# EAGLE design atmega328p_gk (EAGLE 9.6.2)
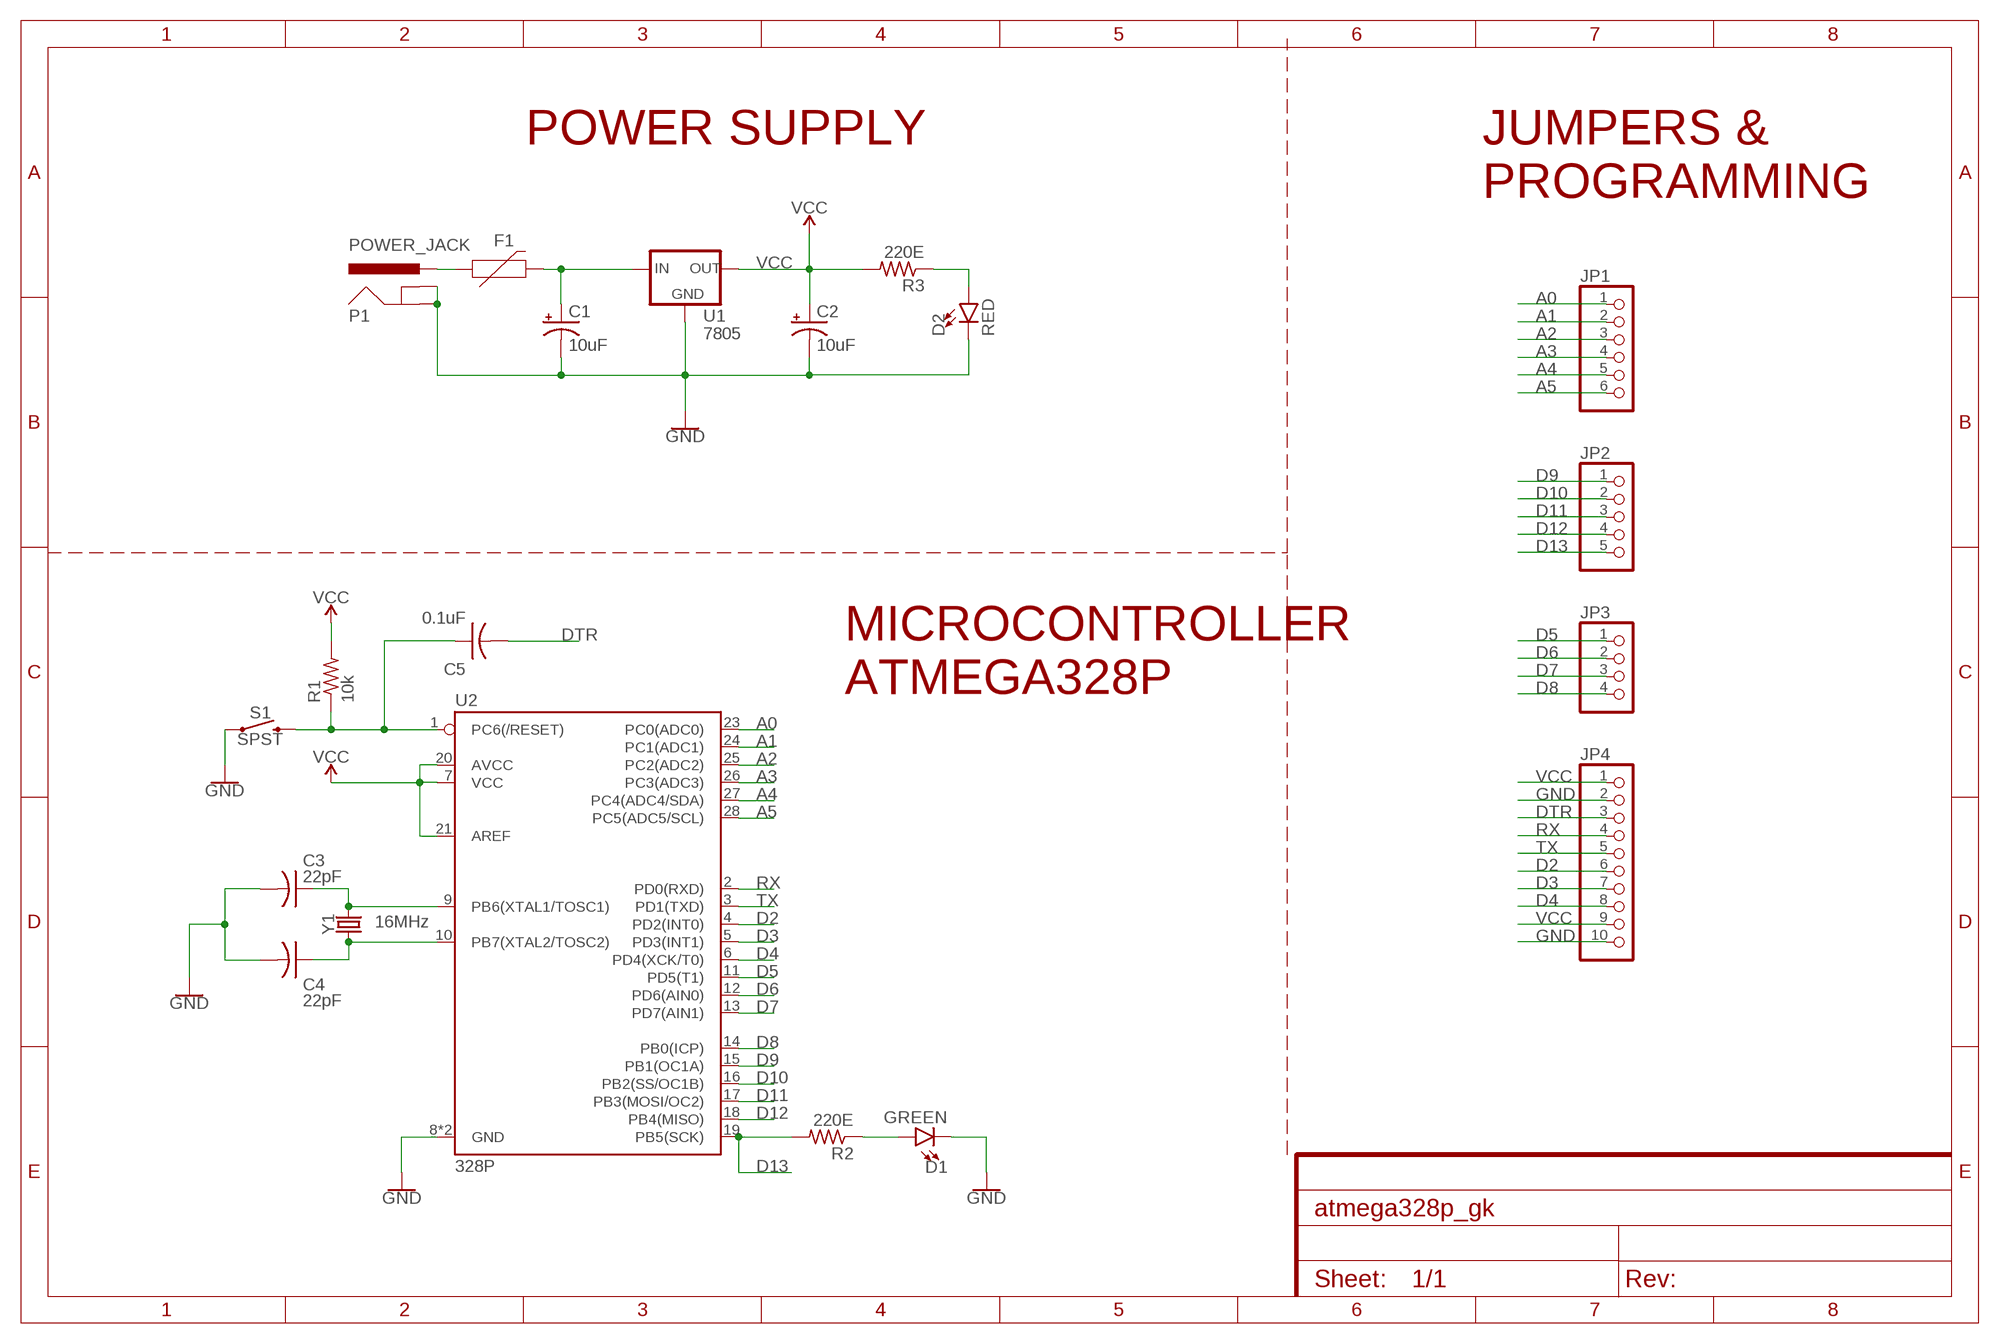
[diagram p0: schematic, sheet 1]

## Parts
C1  10uF  CPOL-USE2,5-6E  [E2,5-6E]
C2  10uF  CPOL-USE2,5-6E  [E2,5-6E]
C3  22pF  C-US025-024X044  [C025-024X044]
C4  22pF  C-US025-024X044  [C025-024X044]
C5  0.1uF  C-US025-024X044  [C025-024X044]
D1  GREEN  LED-GREEN0603  [LED-0603]
D2  RED  LED-RED0603  [LED-0603]
F1  PPTC_16V_2.5A  [1812]
JP1  PINHD-1X6  [1X06]
JP2  PINHD-1X5  [1X05]
JP3  PINHD-1X4  [1X04]
JP4  PINHD-1X10  [1X10]
P1  POWER_JACK  POWER_JACKPTH_LOCK  [POWER_JACK_PTH_LOCK]
R1  10k  R-US_0204/7  [0204/7]
R2  220E  R-US_0204/7  [0204/7]
R3  220E  R-US_0204/7  [0204/7]
S1  SPST  MOMENTARY-SWITCH-SPST-PTH-6.0MM  [TACTILE_SWITCH_PTH_6.0MM]
U1  7805  78XXS  [78XXS]
U2  328P  ATMEGA328P_PDIP  [DIP28]
Y1  16MHz  CRYSTAL-16MHZPTH-HC49US  [HC49US]

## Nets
A0: JP1.1 U2.23(PC0(ADC0))
A1: JP1.2 U2.24(PC1(ADC1))
A2: JP1.3 U2.25(PC2(ADC2))
A3: JP1.4 U2.26(PC3(ADC3))
A4: JP1.5 U2.27(PC4(ADC4/SDA))
A5: JP1.6 U2.28(PC5(ADC5/SCL))
D2: JP4.6 U2.4(PD2(INT0))
D3: JP4.7 U2.5(PD3(INT1))
D4: JP4.8 U2.6(PD4(XCK/T0))
D5: JP3.1 U2.11(PD5(T1))
D6: JP3.2 U2.12(PD6(AIN0))
D7: JP3.3 U2.13(PD7(AIN1))
D8: JP3.4 U2.14(PB0(ICP))
D9: JP2.1 U2.15(PB1(OC1A))
D10: JP2.2 U2.16(PB2(SS/OC1B))
D11: JP2.3 U2.17(PB3(MOSI/OC2))
D12: JP2.4 U2.18(PB4(MISO))
D13: JP2.5 R2.2 U2.19(PB5(SCK))
DTR: C5.2 JP4.3
GND: C1.- C2.- C3.2 C4.2 D1.C D2.C JP4.2 JP4.10 P1.GND P1.GNDBREAK S1.1 U1.GND U2.8(GND) U2.22(GND)
N$1: C1.+ F1.2 U1.IN
N$2: C3.1 U2.9(PB6(XTAL1/TOSC1)) Y1.2
N$3: C4.1 U2.10(PB7(XTAL2/TOSC2)) Y1.1
N$5: C5.1 R1.1 S1.3 U2.1(PC6(/RESET))
N$6: D2.A R3.1
N$7: D1.A R2.1
N$8: F1.1 P1.PWR
RX: JP4.4 U2.2(PD0(RXD))
TX: JP4.5 U2.3(PD1(TXD))
VCC: C2.+ JP4.1 JP4.9 R1.2 R3.2 U1.OUT U2.7(VCC) U2.20(AVCC) U2.21(AREF)

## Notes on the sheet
- POWER SUPPLY
- JUMPERS & 
  PROGRAMMING
- MICROCONTROLLER 
  ATMEGA328P

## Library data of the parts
C1 C2 = rcl:CPOL-US: POLARIZED CAPACITOR, American symbol; SPICEPREFIX: C
C3-C5 = rcl:C-US: CAPACITOR, American symbol; SPICEPREFIX: C
D1 = SparkFun-LED:LED-GREEN: Green SMD LED; PROD_ID: DIO-00821
D2 = SparkFun-LED:LED-RED: Red SMD LED; PROD_ID: DIO-00819
F1 = SparkFun-Fuses:PPTC: Resettable Fuse PPTC; PROD_ID: RES-14390; VALUE: 16V/2.5A(5A TRIP)
JP1 = pinhead:PINHD-1X6: PIN HEADER
JP2 = pinhead:PINHD-1X5: PIN HEADER
JP3 = pinhead:PINHD-1X4: PIN HEADER
JP4 = pinhead:PINHD-1X10: PIN HEADER
P1 = SparkFun-Connectors:POWER_JACK: Power Jack Connector This is the standard 5.5mm barrel jack for power. The PTH is the most common, proven, reliable, footprint. The Slot footprint only works if the mill layer is transmitted to the PCB fab house so be warned. Here are the connectors we sell at SparkFun: DC Barrel Power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; PROD_ID: CONN-08197; SF_ID: PRT-00119
R1-R3 = rcl:R-US_: RESISTOR, American symbol; SPICEPREFIX: R
S1 = SparkFun-Switches:MOMENTARY-SWITCH-SPST: Momentary Switch (Pushbutton) - SPST; PROD_ID: SWCH-08441; SF_SKU: COM-00097
U1 = v-reg:78XXS: VOLTAGE REGULATOR
U2 = SparkFun-IC-Microcontroller:ATMEGA328P_PDIP: Atmel 328P Through hole ATMEGA328P uC used in the Arduino 32kb flash, 1k EEPROM, 2k SRAM Datasheet SparkFun Products Storefront component: AVR 28 Pin 20MHz 32K 6A/D - ATMega328P (COM-09061) SparkFun Simon Says - Through-Hole Soldering Kit (KIT-10547) SparkFun Learn to Solder - Simon Says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; PROD_ID: IC-09136
Y1 = SparkFun-Clocks:CRYSTAL-16MHZ: 16MHz Crystal; PROD_ID: XTAL-08181; SF_ID: COM-00536

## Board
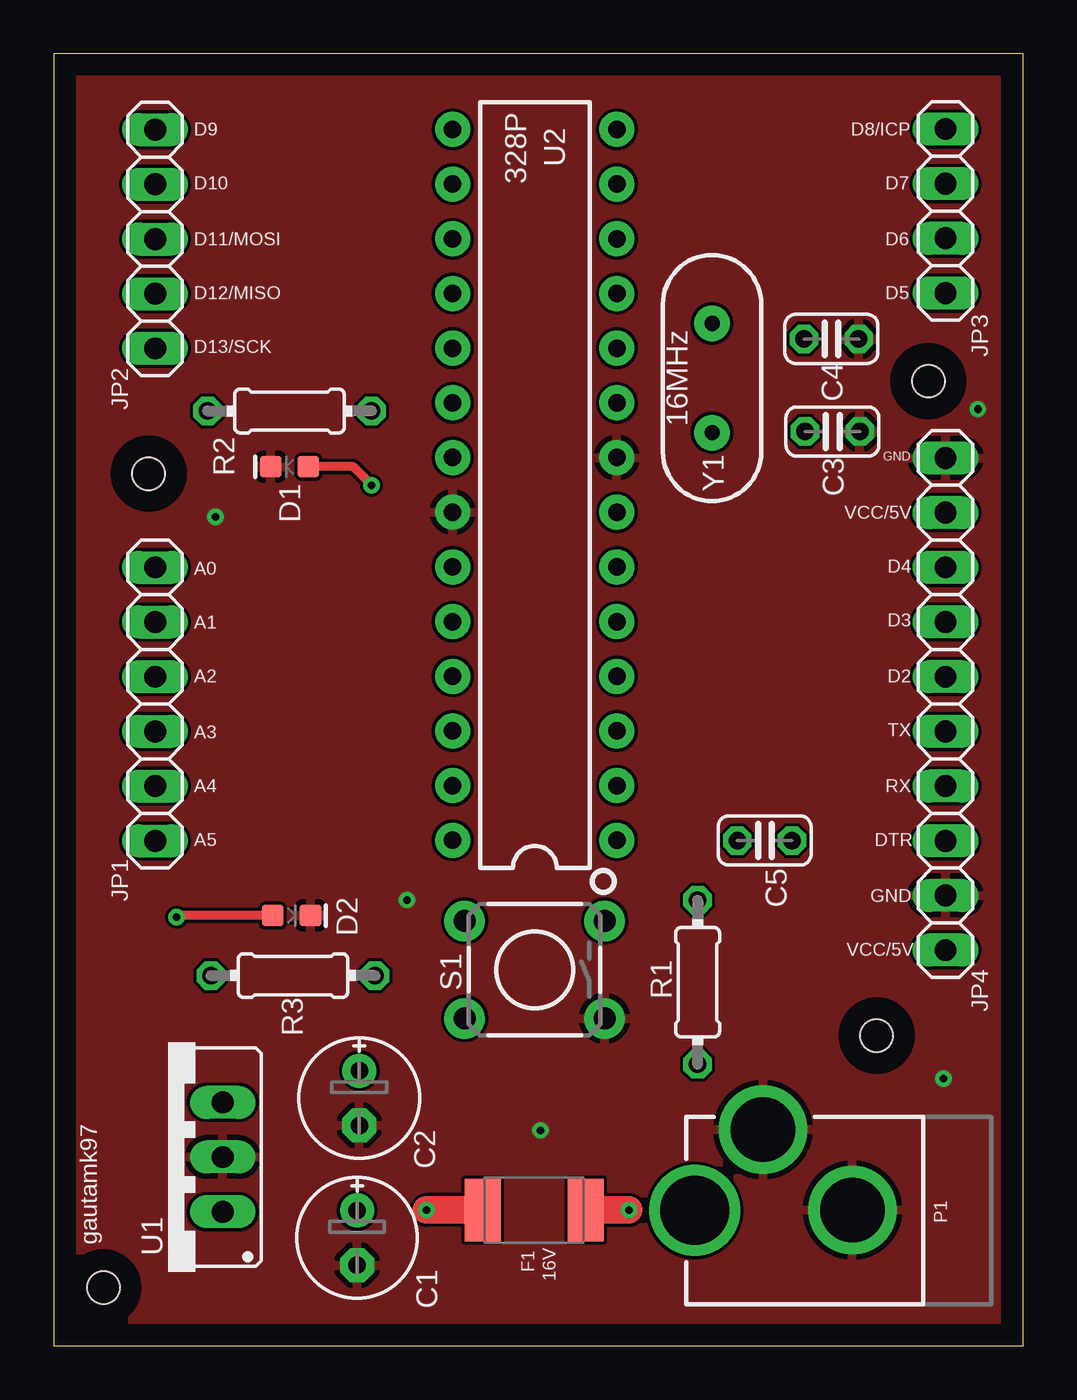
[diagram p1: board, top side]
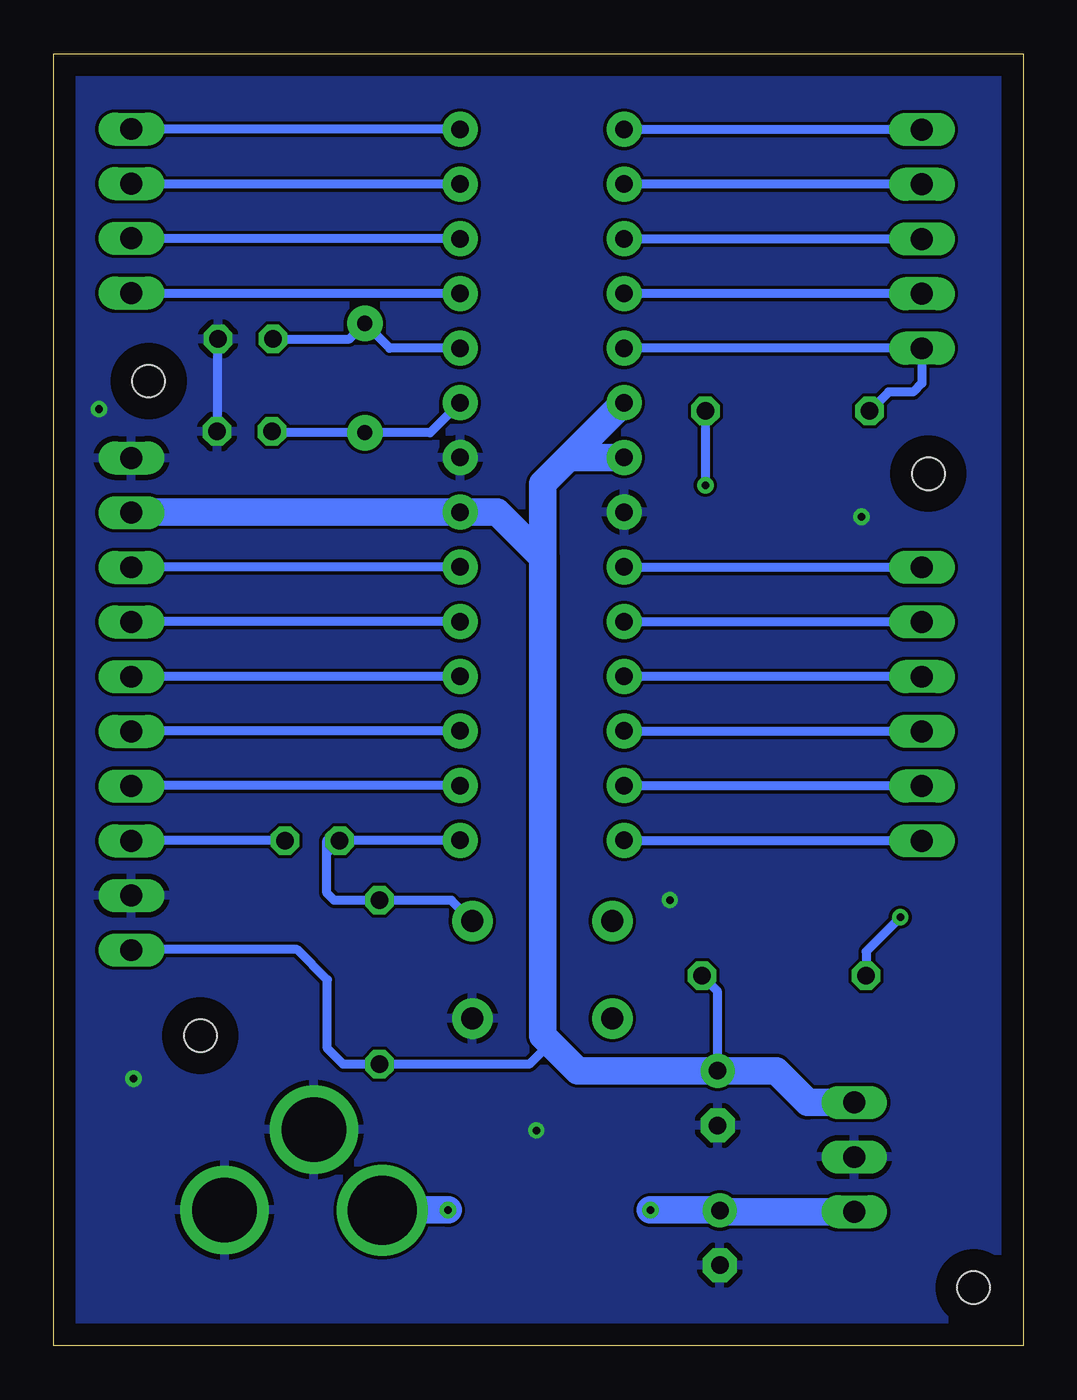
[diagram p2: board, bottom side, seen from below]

Size 45 x 60 mm. Coordinates in mm from the lower left corner, seen from the top.
Outline: 0,0 45,0 45,60 0,60 0,0
Copper layers (1*16): Top 0.035mm / dielectric 1.5mm / Bottom 0.035mm
Design rules "default": minimum track width 6mil, minimum drill 0.35mm, track to track 6mil, track to pad 6mil, pad to pad 6mil, via to via 6mil, smd to smd 6mil, copper to edge 40mil, drill to drill 6mil, minimum pad ring 10mil, minimum via ring 8mil, stop-mask expansion 4mil, vias tented up to drill 0mil, thermal gap 10mil
Holes 1.5 mm at 38.2,14.4 2.3,2.7 4.4,40.5 40.6,44.8

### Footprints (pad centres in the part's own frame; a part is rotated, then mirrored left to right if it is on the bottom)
E2,5-6E = drill 0.813 pad 1.575: + -1.27,0 | drill 0.813 pad 1.575 octagon: - 1.27,0
C025-024X044 = drill 0.813 octagon: 1 -1.27,0; 2 1.27,0
LED-0603 = smd 1 x 1: A -0.877,0; C 0.877,0
1812 = smd 1.676 x 2.896: 1 -2.388,0; 2 2.388,0
1X06 = drill 1.016 long: 1 -6.35,0; 2 -3.81,0; 3 -1.27,0; 4 1.27,0; 5 3.81,0; 6 6.35,0
1X05 = drill 1.016 long: 1 -5.08,0; 2 -2.54,0; 3 0,0; 4 2.54,0; 5 5.08,0
1X04 = drill 1.016 long: 1 -3.81,0; 2 -1.27,0; 3 1.27,0; 4 3.81,0
1X10 = drill 1.016 long: 1 -11.43,0; 2 -8.89,0; 3 -6.35,0; 4 -3.81,0; 5 -1.27,0; 6 1.27,0; 7 3.81,0; 8 6.35,0; 9 8.89,0; 10 11.43,0
POWER_JACK_PTH_LOCK = drill 2.997 pad 4.115: GND 0.025,6.557; GNDBREAK 3.762,10.7 | drill 3.2 pad 4.115: PWR 0,13.878
0204/7 = drill 0.813 octagon: 1 -3.81,0; 2 3.81,0
TACTILE_SWITCH_PTH_6.0MM = drill 1.016 pad 1.88: 1 -3.251,2.261; 2 3.251,2.261; 3 -3.251,-2.261; 4 3.251,-2.261
78XXS = drill 1.016 long: GND 0,-2.54; IN -2.54,-2.54; OUT 2.54,-2.54
DIP28 = drill 0.813 pad 1.626: 1 -16.51,-3.81; 2 -13.97,-3.81; 3 -11.43,-3.81; 4 -8.89,-3.81; 5 -6.35,-3.81; 6 -3.81,-3.81; 7 -1.27,-3.81; 8 1.27,-3.81; 9 3.81,-3.81; 10 6.35,-3.81; 11 8.89,-3.81; 12 11.43,-3.81; 13 13.97,-3.81; 14 16.51,-3.81; 15 16.51,3.81; 16 13.97,3.81; 17 11.43,3.81; 18 8.89,3.81; 19 6.35,3.81; 20 3.81,3.81; 21 1.27,3.81; 22 -1.27,3.81; 23 -3.81,3.81; 24 -6.35,3.81; 25 -8.89,3.81; 26 -11.43,3.81; 27 -13.97,3.81; 28 -16.51,3.81
HC49US = drill 0.7 pad 1.651: 1 -2.54,0; 2 2.54,0

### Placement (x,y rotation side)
C1  14.08,5.01 270 top
C2  14.18,11.5 270 top
C3  36.15,42.46 0 top
C4  36.1,46.76 0 top
C5  33,23.46 0 top
D1  10.94,40.82 180 top
D2  11.04,19.98 0 top
F1  22.3,6.3 180 top
JP1  4.7,29.8 270 top
JP2  4.7,51.4 270 top
JP3  41.4,52.7 90 top
JP4  41.4,29.8 90 top
P1  43.63,6.28 90 top
R1  29.89,16.88 270 top
R2  10.94,43.41 180 top
R3  11.1,17.19 0 top
S1  22.32,17.46 180 top
U1  5.3,8.76 90 top
U2  22.33,39.98 90 top
Y1  30.56,44.94 270 top

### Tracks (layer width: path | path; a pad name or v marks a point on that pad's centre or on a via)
A0
  Bottom 0.406: JP1.1 18.5,36.15 U2.23
A1
  Bottom 0.406: JP1.2 18.5,33.61 U2.24
A2
  Bottom 0.406: JP1.3 18.5,31.07 U2.25
A3
  Bottom 0.406: JP1.4 18.5,28.53 U2.26
A4
  Bottom 0.406: JP1.5 18.5,25.99 U2.27
A5
  Bottom 0.406: JP1.6 18.5,23.45 U2.28
D2
  Bottom 0.406: U2.4 41.38,31.09 JP4.6
D3
  Bottom 0.406: U2.5 41.38,33.63 JP4.7
D4
  Bottom 0.406: U2.6 41.38,36.17 JP4.8
D5
  Bottom 0.406: U2.11 41.38,48.87 JP3.1
D6
  Bottom 0.406: U2.12 41.38,51.41 JP3.2
D7
  Bottom 0.406: U2.13 41.38,53.95 JP3.3
D8
  Bottom 0.406: U2.14 41.38,56.49 JP3.4
D9
  Bottom 0.406: JP2.1 U2.15
D10
  Bottom 0.406: JP2.2 U2.16
D11
  Bottom 0.406: JP2.3 U2.17
D12
  Bottom 0.406: JP2.4 U2.18
D13
  Bottom 0.406: U2.19 JP2.5 4.7,44.7 5.1,44.3 6.24,44.3 R2.2
DTR
  Bottom 0.406: C5.2 JP4.3
GND  (via drill 0.35)
  Bottom 0.406: C4.2 37.42,46.71 C3.2
  other vias: 7.5,38.5 42.9,43.5 41.3,12.4 22.6,10 16.4,20.7
  pour Bottom: 0.1,0 45,0 45,59.9 0.1,59.9
  pour Top: 0.1,60 0.1,0 45.1,0 45.1,60
N$1  (via drill 0.35)
  Top 1.27: F1.2 v17.3,6.3
  Bottom 1.27: U1.IN 14.02,6.22 C1.+ 14.1,6.3 v17.3,6.3
N$2
  Bottom 0.406: U2.9 27.53,42.4 Y1.2 34.82,42.4 C3.1
N$3
  Bottom 0.406: U2.10 29.41,46.33 Y1.1 31.28,46.76 C4.1
N$5
  Bottom 0.406: U2.1 32.32,23.47 32.32,22.87 | 32.32,22.87 C5.1 | 32.32,22.87 32.32,21.02 31.99,20.69 R1.1 26.54,20.69 S1.3
N$6  (via drill 0.35)
  Top 0.406: D2.A 5.78,19.98 v5.7,19.9
  Bottom 0.406: v5.7,19.9 7.29,18.31 R3.1
N$7  (via drill 0.35)
  Top 0.406: v14.75,39.96 13.89,40.82 D1.A
  Bottom 0.406: R2.1 v14.75,39.96
N$8  (via drill 0.35)
  Top 1.27: F1.1 v26.7,6.3
  Bottom 1.27: v26.7,6.3 29.73,6.3 P1.PWR
RX
  Bottom 0.406: U2.2 41.38,26.01 JP4.4
TX
  Bottom 0.406: U2.3 41.38,28.55 JP4.5
VCC
  Bottom 0.406: R3.2 14.2,16.48 14.2,12.79 C2.+ | 22.3,14.4 22.3,13.7 22.93,13.07 R1.2 31.57,13.07 32.3,13.8 32.3,17 33.7,18.4 41.37,18.4 JP4.1
  Bottom 1.27: U1.OUT 10,11.3 11.47,12.77 C2.+ 20.67,12.77 22.3,14.4 22.3,36.6 | U2.20 21.07,41.27 | 22.3,36.6 22.3,40.03 21.07,41.27 | U2.21 21.05,41.25 21.07,41.27 | 22.3,36.6 24.41,38.71 U2.7 41.38,38.71 JP4.9

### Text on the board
tNames: D9 | D8/ICP | D10 | D7 | D11/MOSI | D6 | D12/MISO | D5 | D13/SCK | GND | VCC/5V | A0 | D4 | A1 | D3 | A2 | D2 | A3 | TX | A4 | RX | A5 | DTR | GND | VCC/5V | gautamk97 | 16V

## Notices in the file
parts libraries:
SparkFun-Connectors: Licensing: Creative Commons ShareAlike 4.0 International - https://creativecommons.org/licenses/by-sa/4.0
